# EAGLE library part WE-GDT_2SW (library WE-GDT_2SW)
SMD Gate Drive Transformer WE-GDT - small form factor EP5 - 1 or 2 secondary windings - 4 different turn rations - 1500VDC insulation test voltage - operating voltage up to 80V -- Gate Drive -- Signal -- Power -- Synchronous Flyback
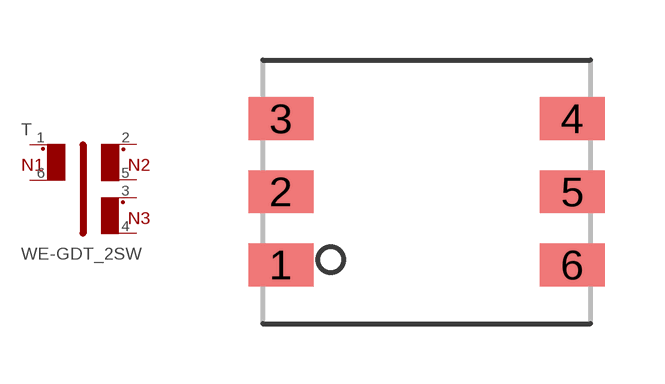
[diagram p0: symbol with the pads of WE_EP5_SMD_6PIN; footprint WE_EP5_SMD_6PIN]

Designator prefix T

## WE-GDT_2SW_760301103, WE-GDT_2SW-760301103_760301103 (MPN: 760301103; OC_FARNELL: 2114313; OC_NEWARK: 06W1238; PACKAGE: EP5; SUPPLIER: Wuerth Elektronik)  [WE_EP5_SMD_6PIN]
1  1  pas
2  3  pas
3  5  pas
4  6  pas
5  4  pas
6  2  pas

## WE-GDT_2SW_760301104, WE-GDT_2SW-760301104_760301104 (MPN: 760301104; OC_FARNELL: 2114314; OC_NEWARK: 06W1239; PACKAGE: EP5; SUPPLIER: Wuerth Elektronik)  [WE_EP5_SMD_6PIN]
Pads as for WE_EP5_SMD_6PIN

## WE-GDT_2SW_760301105, WE-GDT_2SW-760301105_760301105 (MPN: 760301105; OC_FARNELL: 2114315; OC_NEWARK: 06W1240; PACKAGE: EP5; SUPPLIER: Wuerth Elektronik)  [WE_EP5_SMD_6PIN]
Pads as for WE_EP5_SMD_6PIN

## Footprint WE_EP5_SMD_6PIN (pad centres in mm)
Transformer, EP5 SMD 6 Pin
smd 1.63 x 1.07: 1 -3.645,-1.83; 2 -3.645,0; 3 -3.645,1.83; 4 3.645,1.83; 5 3.645,0; 6 3.645,-1.83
